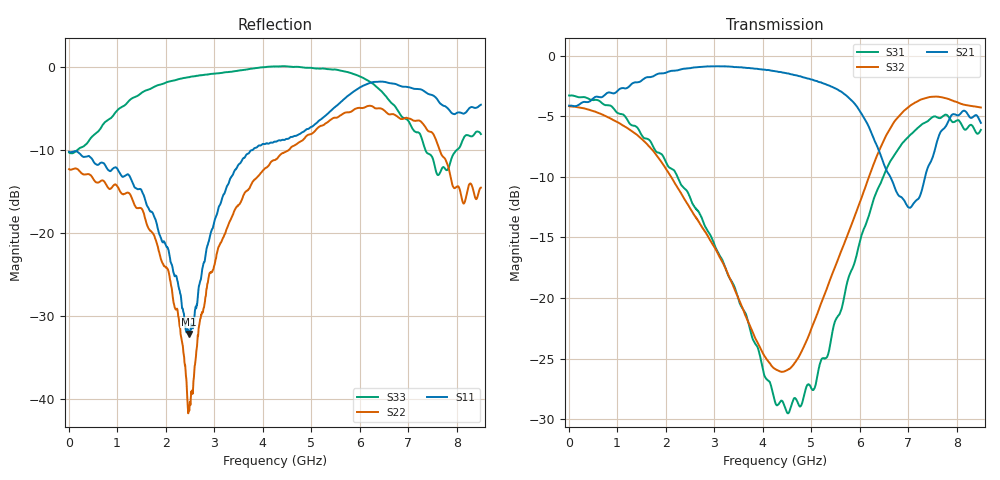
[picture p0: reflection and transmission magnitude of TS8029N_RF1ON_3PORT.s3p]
!Created with skrf (http://scikit-rf.org).
# GHz S RI R 50.0
!freq ReS11 ImS11 ReS12 ImS12 ReS13 ImS13
! ReS21 ImS21 ReS22 ImS22 ReS23 ImS23
! ReS31 ImS31 ReS32 ImS32 ReS33 ImS33
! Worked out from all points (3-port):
!   1601 points, 10 MHz to 8.5 GHz, reference 50 ohm
!   strongest paths, dB at 10 MHz, 2.132 GHz, 4.255 GHz, 6.378 GHz, 8.5 GHz:
!     S21: -4.1, -1.2, -1.3, -7.6, -5.5
!     S32: -4.2, -10.1, -25.9, -8.1, -4.3
!     S31: -3.3, -9.3, -28.6, -11.0, -6.1
!   lowest |S11| = -32.1 dB at 2.472 GHz (marker M1), VSWR 1.05, Z = 47.7 + j0.643 ohm
!   |S11| at or under -10 dB: start of sweep to 3.76 GHz
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0.01  -0.3107 0.00374  0.623 -0.000181  0.6863 -0.00638
      0.6229 -0.0002  -0.2436 0.0027  0.6192 -0.00695
      0.6861 -0.00652  0.6194 -0.00692  -0.3067 0.00999
1.023494  -0.1748 0.1629  0.714 -0.1068  0.3497 -0.4618
          0.714 -0.1069  -0.0932 0.1634  0.2786 -0.4507
          0.3498 -0.4618  0.2789 -0.4511  0.3017 0.4705
2.0476  -0.0281 0.076  0.7375 -0.4404  -0.065 -0.3451
        0.7374 -0.4401  0.0431 0.0427  -0.1538 -0.2943
        -0.0651 -0.3448  -0.1535 -0.2943  0.8035 -0.1531
2.4721  -0.0239 0.00674  0.6612 -0.5942  -0.1349 -0.2338
        0.6614 -0.594  0.00525 -0.00715  -0.1792 -0.1607
        -0.1345 -0.2337  -0.1795 -0.161  0.7284 -0.4817
3.092931  -0.0964 -0.1062  0.4734 -0.7719  -0.1197 -0.0942
          0.4732 -0.7719  -0.0813 -0.0171  -0.1477 -0.0288
          -0.1201 -0.0941  -0.1476 -0.0285  0.3058 -0.8685
4.255  -0.3204 -0.1581  -0.0197 -0.864  -0.0326 -0.0181
       -0.0199 -0.8634  -0.276 0.0176  -0.0183 0.0475
       -0.0327 -0.018  -0.0184 0.0475  -0.5206 -0.8689
5.284413  -0.5076 -0.00773  -0.3785 -0.6653  -0.0516 0.0221
          -0.3782 -0.6663  -0.2064 0.4076  0.0432 0.0951
          -0.0517 0.0221  0.0433 0.0949  -0.9794 -0.0665
6.409338  -0.5427 0.6164  -0.3526 -0.1914  0.1638 0.2412
          -0.3521 -0.192  0.1427 0.5481  0.3933 0.1117
          0.1637 0.2412  0.3936 0.1111  -0.428 0.5983
7.507731  0.0187 0.6783  -0.0919 -0.3707  0.4551 -0.326
          -0.0912 -0.3711  0.4003 -0.000445  0.1988 -0.6485
          0.4557 -0.3247  0.1982 -0.6478  0.1443 0.2432
8.5  0.1163 0.5843  -0.3818 -0.3656  -0.0153 -0.4945
     -0.3822 -0.3655  0.1596 0.1002  -0.3925 -0.4695
     -0.0154 -0.4945  -0.3924 -0.4698  0.1975 0.3437
